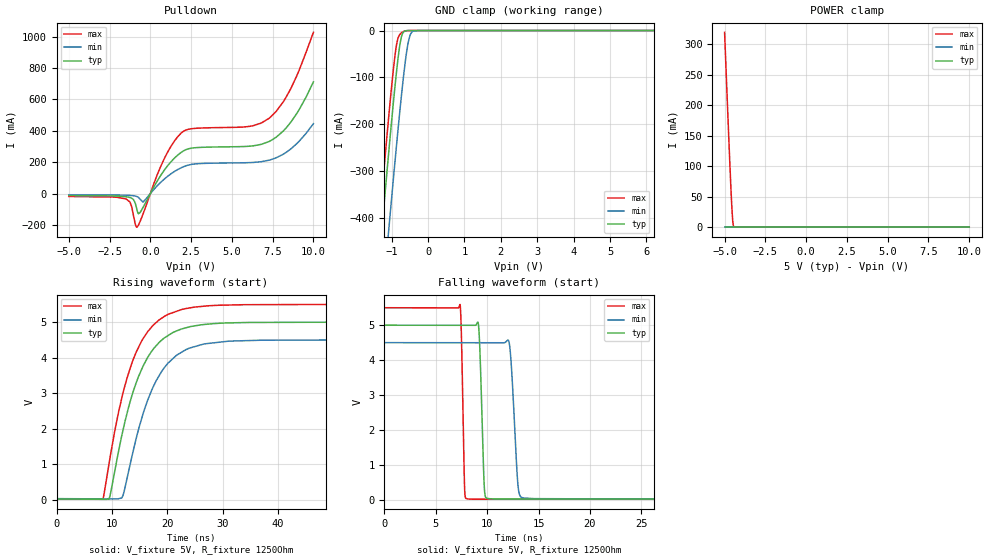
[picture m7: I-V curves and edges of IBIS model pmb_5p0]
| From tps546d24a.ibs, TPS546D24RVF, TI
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|   pmb_5p0 Model
[Model]   pmb_5p0
Model_type   I/O_open_drain
Polarity   Inverting
Enable   Active-High
Vinl = 0.8
Vinh = 1.35
Vmeas = 2.5
Vref = 5
Cref = 2pF
Rref = 1250
|   typ   min   max
C_comp   3.145pF   2.949pF   3.248pF
|C_comp_pull_down   3.578pF   3.433pF   4.184pF
|  Where Nom  PVT is Nominal Process, 5.0V,   25C
|   Fast PVT is Strong Process,  5.5V,  -40C
|   Slow PVT is Weak Process,   4.5V,  150C
[Voltage Range]   5   4.5   5.5
|Junction Temperature
[Temperature Range]   25   150   -40
[Pullup Reference]   5   4.5   5.5
[Pulldown Reference]   0   0   0
[Power Clamp Reference]   5   4.5   5.5
[GND Clamp Reference]   0   0   0
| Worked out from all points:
|   slope of the pulldown table from 0 to 0.75 V, typ, clamps not added: 5.63 ohm
|   GND clamp passes 1 mA (typ) near -0.63 V on its own axis
|   falling waveform, V_fixture 5V, R_fixture 1250Ohm: 20-80 % time 309ps typ, 477ps min, 223ps max; typ from 5 V to 0.02 V
|   rising waveform, V_fixture 5V, R_fixture 1250Ohm: 20-80 % time 5.67ns typ, 5.76ns min, 5.57ns max; typ from 0.02 V to 5 V
[Pulldown]
|   Voltage   I(typ)   I(min)   I(max)
-5V       -12.26mA   -7.486mA   -17.94mA
-1.49V    -19.44mA   -9.962mA   -33.56mA
-1.25V    -24.39mA   -11.19mA   -53.15mA
-815mV    -104.1mA   -19mA      -212.9mA
-440mV    -86.52mA   -52.37mA   -128mA
640mV     116.4mA    72.13mA    174.1mA
1.69V     246.4mA    154mA      363.7mA
2.335V    285.5mA    181.9mA    409.8mA
6.1V      302.1mA    197.5mA    428.5mA
7.27V     331.4mA    212.7mA    478.9mA
8.56V     447.8mA    280.3mA    658.2mA
10V       711.4mA    445.4mA    1.027A
[GND Clamp]
|   Voltage   I(typ)   I(min)   I(max)
-5V       -3.907A    -4.042A    -3.852A
-1.445V   -579.9mA   -745.6mA   -503.2mA
-1.25V    -405.6mA   -572.2mA   -328.3mA
-1.07V    -249.3mA   -415mA     -173.3mA
-965mV    -162.2mA   -325.4mA   -90.63mA
-860mV    -82.2mA    -238.3mA   -27.18mA
-770mV    -27.77mA   -167mA     -7.827mA
-665mV    -2.334mA   -90.77mA   -1.824mA
-545mV    -100.4uA   -24.85mA   -117.5uA
-485mV    -20.07uA   -8.077mA   -20.48uA
-410mV    -2.141uA   -1.291mA   -1.428uA
10V       0A         0A         0A
[POWER Clamp]
|   Voltage   I(typ)   I(min)   I(max)
-5V       2.908nA    41.44nA    319.5mA
-4.865V   0A         3.588nA    227.5mA
-4.745V   0A         1.993nA    147.6mA
-4.655V   0A         852.1pA    90.14mA
-4.595V   0A         117.1pA    54.37mA
-4.55V    0A         0A         30.44mA
-4.505V   0A         0A         11.8mA
-4.475V   0A         0A         4.424mA
-4.43V    0A         0A         613.5uA
10V       0A         0A         0A
[Ramp]
R_load = 1250
|   typ   min   max
dV/dt_r   2.98827/5.68027e-09   2.68289/5.76019e-09   3.29141/5.55631e-09
dV/dt_f   2.98827/3.09249e-10   2.68289/4.77213e-10   3.29141/2.23455e-10
[Falling Waveform]
V_fixture = 5V
V_fixture_min = 4.5V
V_fixture_max = 5.5V
R_fixture = 1250Ohm
C_fixture = 0F
|   Time   V(typ)   V(min)   V(max)
0s        5V         4.5V       5.5V
7.357ns   4.997V     4.498V     5.593V
7.828ns   4.997V     4.498V     190mV
8.496ns   4.997V     4.498V     18.21mV
9.191ns   4.885V     4.498V     18.2mV
9.793ns   134.5mV    4.498V     18.2mV
10.62ns   24.86mV    4.497V     18.19mV
12.11ns   24.85mV    4.54V      18.18mV
14.49ns   24.82mV    34.89mV    18.16mV
500ns     19.55mV    28.49mV    14.31mV
[Rising Waveform]
V_fixture = 5V
V_fixture_min = 4.5V
V_fixture_max = 5.5V
R_fixture = 1250Ohm
C_fixture = 0F
|   Time   V(typ)   V(min)   V(max)
0s        19.55mV    28.49mV    14.31mV
8.354ns   9.657mV    21.58mV    13.18mV
9.611ns   78.94mV    20.54mV    1.134V
11.79ns   1.81V      50.57mV    2.868V
13.39ns   2.815V     1.06V      3.744V
14.78ns   3.458V     1.96V      4.282V
18.04ns   4.346V     3.366V     4.999V
21.67ns   4.754V     4.07V      5.308V
27.36ns   4.947V     4.401V     5.463V
500ns     5V         4.5V       5.5V
